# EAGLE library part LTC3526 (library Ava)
Linear LTC3526 http://cds.linear.com/docs/en/datasheet/3526bfd.pdf Anthony Stirk March 2014
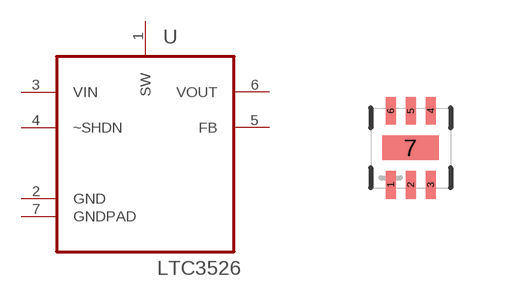
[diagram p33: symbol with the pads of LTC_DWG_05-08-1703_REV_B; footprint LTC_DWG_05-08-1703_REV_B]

Designator prefix -

## LTC3526  [LTC_DWG_05-08-1703_REV_B]
1  SW  in
2  GND  pas
3  VIN  pwr
4  ~SHDN  pas
5  FB  in
6  VOUT  out
7  GNDPAD  pas

## Footprint LTC_DWG_05-08-1703_REV_B (pad centres in mm)
smd 0.25 x 0.7: 1 -0.5,-0.925; 2 0,-0.925; 3 0.5,-0.925; 4 0.5,0.925; 5 0,0.925; 6 -0.5,0.925
smd 1.42 x 0.61: 7 0,0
